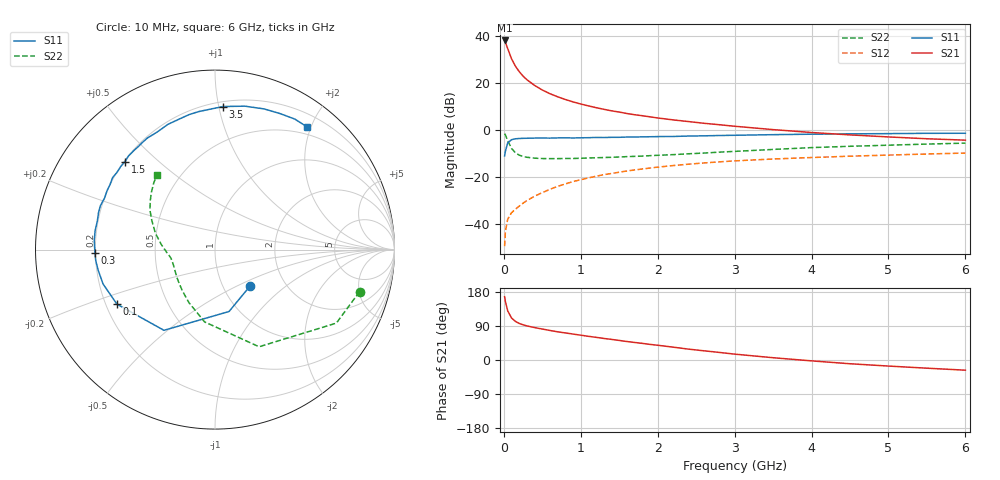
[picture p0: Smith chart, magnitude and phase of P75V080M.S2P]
! SIEMENS Small Signal Semiconductors
! BFP196
! Si NPN RF Bipolar Junction Transistor in SOT143
! VCE = 5 V  IC = 80 mA
! Common Emitter S-Parameters:  May  1996
# GHz  S  MA  R  50
!  f  S11  S21  S12  S22
! GHz  MAG  ANG  MAG  ANG  MAG  ANG  MAG  ANG
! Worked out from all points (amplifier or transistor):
!   36 points, 10 MHz to 6 GHz, reference 50 ohm
!   highest |S21| = 38.1 dB at 10 MHz (marker M1)
!   |S21| within 3 dB of that: start of sweep to 45.06 MHz
!   unconditionally stable (mu >= 1): 395.8 MHz to 4.494 GHz
!   at 250 MHz: K = 0.89, MSG = 27.0 dB, |S12| = -31.1 dB
!   at 1.4 GHz: K = 1.08, MAG = 11.5 dB, |S12| = -18.5 dB
!   at 6 GHz: K = 0.98, MSG = 2.7 dB, |S12| = -9.8 dB
!   S11 on the Smith chart (normalised r, x): 10 MHz: 1.34, -0.59; 100 MHz: 0.25, -0.24; 300 MHz: 0.20, -0.01; 1.5 GHz: 0.20, +0.39; 3.5 GHz: 0.23, +1.03; 6 GHz: 0.38, +1.94
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0.01  0.2814 -45.6  80.33 166.9  0.0034 75.5  0.8389 -16.2
0.02  0.3536 -77.2  73.92 154.4  0.0069 69.8  0.7906 -31.2
0.05  0.5321 -122.3  54.01 129.8  0.0127 54.2  0.5944 -65.6
0.1  0.6252 -150.9  32.79 110.8  0.0175 50.5  0.407 -98.2
0.15  0.6524 -162.9  22.87 101.9  0.0208 51.6  0.3288 -116.3
0.2  0.6607 -169.8  17.47 96.5  0.0241 55.8  0.2933 -128.2
0.25  0.6672 -174.7  14 92.8  0.0279 57.7  0.2735 -137.2
0.3  0.6694 -178.3  11.75 90.0  0.0317 60.7  0.2639 -143.0
0.4  0.675 175.4  8.879 85.5  0.0393 63.2  0.2526 -151.6
0.5  0.6761 170.8  7.103 81.7  0.0468 64.4  0.2481 -157.1
0.6  0.6745 166.4  5.922 77.9  0.0551 64.7  0.2467 -160.9
0.7  0.681 162.3  5.096 74.4  0.0635 64.7  0.2472 -163.8
0.8  0.6837 159.0  4.46 71.4  0.0716 63.9  0.2488 -166.1
0.9  0.6791 155.1  3.967 68.4  0.0803 63.2  0.2489 -168.2
1.1  0.688 148.3  3.264 62.5  0.0961 61.1  0.2547 -171.2
1.5  0.7012 135.6  2.414 51.6  0.1271 55.9  0.2675 -176.1
2.2  0.7303 116.0  1.645 33.9  0.1759 45.4  0.3002 174.6
2.8  0.766 100.8  1.299 20.0  0.2107 36.4  0.3395 165.5
3.5  0.7984 86.8  1.022 6.0  0.2424 26.3  0.3875 155.3
4.5  0.8301 70.8  0.789 -9.9  0.2782 14.2  0.4519 143.0
5.5  0.8523 58.6  0.653 -21.6  0.3096 3.5  0.5032 132.8
6  0.8546 53.2  0.61 -26.9  0.3245 -2.1  0.5276 127.9
